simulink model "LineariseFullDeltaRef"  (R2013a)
settings: Solver=ode23tb  StartTime=0.0  StopTime=2  RelTol=1e-3
InitFcn:
  | SimParam.IC = SM2_InitCondConstrFnc(RawParam,IC);
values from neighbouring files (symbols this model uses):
  N = D(1)+(H4^2+H3^2)/H2^2-(E(1)*H4+F(1)*H3)/H2    [MGD.m]    (also in MGD2.m)
  RawParam = RobotParamGather(ParamLib)    [main_testIdentification3quad.m]    (also in DeltaModelMain_v2.m; main_TimeSimulation.m; MGI.m = y)
  s = -sign(imag(KGZ_fr_tmp))    [LinprogReguliOptimFunc_1.m]    (also in LinprogReguliOptimFunc_2.m; LinprogReguliOptimFunc_1 - Copie.m)
  X = varDefaultValue    [main_OptimModelParam1_subfunc1.m]    (also in main_OptimModelParam2_subfunc1.m; main_testIdentification3bis.m = [180e-6  370e-6         0.00182               0.95          ; main_testIdentification3tris.m = [180e-6 370e-6 0.00182 1 6.65e-3 0.0019 0.01 100  0.073  435; main_testIdentification3_ga_subfunc1.m)
  Y = fft(y(:,i),NFFT)/L    [fft_bis.m]    (also in MGI.m = -sin(phi(i))*x+cos(phi(i))*y)
  Z = z    [MGI.m]
undefined symbols (not defined in the file or in its folder): AxisID, kg, m, rad
libraries: sm_lib x29, SM2_ArmPartsLib x12, SM2_BallJointPartsLib x10, SM2_ForeArmPartsLib x6, nesl_utility x4, SM2_MotorPartsLib x3, SM2_FramePartsLib x1, SM2_ToolPartsLib x1

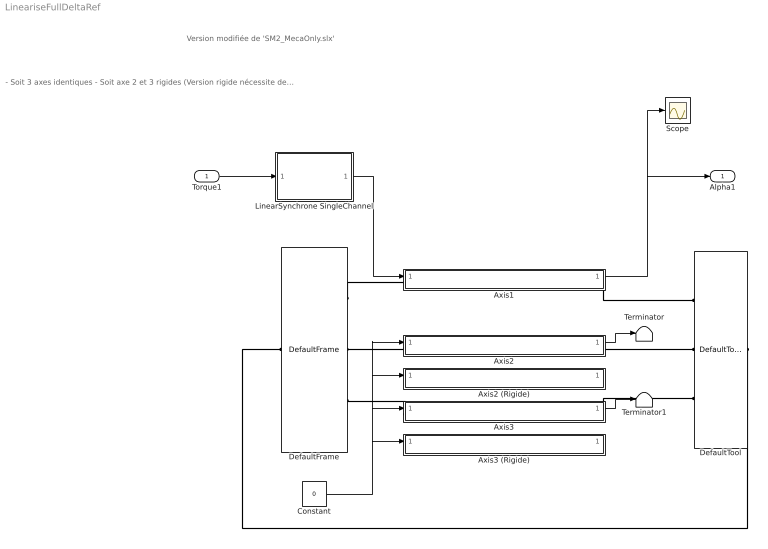
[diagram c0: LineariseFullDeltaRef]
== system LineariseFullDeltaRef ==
  note: - Soit 3 axes identiques - Soit axe 2 et 3 rigides (Version rigide nécessite des blocks non liés au libraries et des fonctions d'initialisaions indépendantes voir "local###_paramInitFnc()")
  note: Version modifiée de 'SM2_MecaOnly.slx'
  Torque1 : Inport
  Axis1 : Subsystem
  Axis2 : Subsystem
  Axis2 (Rigide) : Subsystem  Commented=on
  Axis3 : Subsystem
  Axis3 (Rigide) : Subsystem  Commented=on
  Constant : Constant  Value=0
  DefaultFrame : SM2_FramePartsLib/DefaultFrame
  DefaultTool : SM2_ToolPartsLib/DefaultTool
  LinearSynchrone SingleChannel : Subsystem  InitFcn=SimParam.Driver = driver_ParamInitFnc(RawParam,2);  VariantControl=driverVarLinearSynchrone
  Scope : Scope
  Terminator : Terminator
  Terminator1 : Terminator
  Alpha1 : Outport
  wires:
  Axis1/1(Alpha) -> Scope/1, Alpha1/1
  LinearSynchrone SingleChannel/1(Torque) -> Axis1/1(Torque)
  Torque1/1 -> LinearSynchrone SingleChannel/1(U)
  Axis3/1(Alpha) -> Terminator1/1
  Axis2/1(Alpha) -> Terminator/1
  Constant/1 -> Axis3 (Rigide)/1(Torque), Axis3/1(Torque), Axis2 (Rigide)/1(Torque), Axis2/1(Torque)
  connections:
  DefaultFrame/RConn1 -- Axis1/LConn1
  Axis1/RConn1 -- DefaultTool/RConn1
  DefaultTool/LConn1 -- DefaultFrame/LConn1
  Axis2/LConn1 -- DefaultFrame/RConn2
  Axis2/RConn1 -- DefaultTool/RConn2
  Axis3/LConn1 -- DefaultFrame/RConn3
  Axis3/RConn1 -- DefaultTool/RConn3

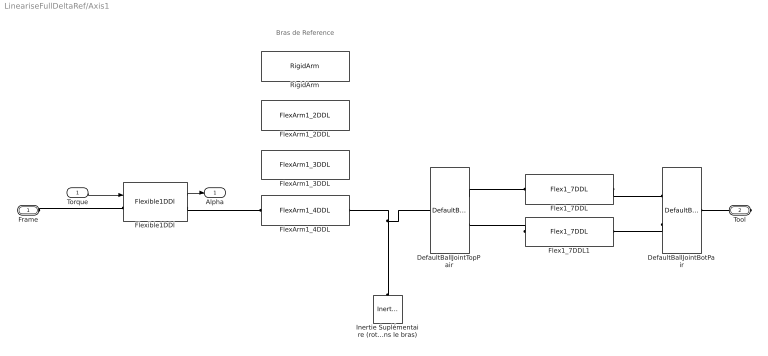
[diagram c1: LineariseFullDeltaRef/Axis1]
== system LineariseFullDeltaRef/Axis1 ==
  note: Bras de Reference
  Torque : Inport
  DefaultBallJointBotPair : SM2_BallJointPartsLib/DefaultBallJointBotPair
  DefaultBallJointTopPair : SM2_BallJointPartsLib/DefaultBallJointTopPair
  Flex1_7DDL : SM2_ForeArmPartsLib/Flex1_7DDL  VariantControl=foreArmVarFlex1_7ddl
  Flex1_7DDL1 : SM2_ForeArmPartsLib/Flex1_7DDL  VariantControl=foreArmVarFlex1_7ddl
  FlexArm1_2DDL : SM2_ArmPartsLib/FlexArm1_2DDL  Commented=on  VariantControl=armVarFlex1_2ddl
  FlexArm1_3DDL : SM2_ArmPartsLib/FlexArm1_3DDL  Commented=on  VariantControl=armVarFlex1_3ddl
  FlexArm1_4DDL : SM2_ArmPartsLib/FlexArm1_4DDL  VariantControl=armVarFlex1_4ddl
  Flexible1DDl : SM2_MotorPartsLib/Flexible1DDl  VariantControl=motorVarFlex1
  Inertie Suplémentaire (rotule déjà inclues dans le bras) : sm_lib/Body Elements/Inertia  InertiaType=Custom  Mass=SimParam.mend+1e-7  MassUnits=kg  CenterOfMass=[0 0 0]  CenterOfMassUnits=m  MomentsOfInertia=SimParam.Iend  MomentsOfInertiaUnits=kg*m^2  ProductsOfInertia=[0 0 0]  ProductsOfInertiaUnits=kg*m^2  BlockFunction=simmechanics.library.body_elements.inertia
  RigidArm : SM2_ArmPartsLib/RigidArm  Commented=on  VariantControl=armVarDefault
  Frame : PMIOPort  Port=1  Side=Left
  Tool : PMIOPort  Port=2  Side=Right
  Alpha : Outport
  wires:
  Torque/1 -> Flexible1DDl/1
  Flexible1DDl/1 -> Alpha/1
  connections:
  Frame/RConn1 -- Flexible1DDl/LConn1
  Flexible1DDl/RConn1 -- FlexArm1_4DDL/LConn1
  Inertie Suplémentaire (rotule déjà inclues dans le bras)/RConn1 -- FlexArm1_4DDL/RConn1 -- DefaultBallJointTopPair/RConn1
  Flex1_7DDL1/LConn1 -- DefaultBallJointTopPair/LConn2
  DefaultBallJointTopPair/LConn1 -- Flex1_7DDL/LConn1
  Flex1_7DDL/RConn1 -- DefaultBallJointBotPair/LConn1
  DefaultBallJointBotPair/LConn2 -- Flex1_7DDL1/RConn1
  Tool/RConn1 -- DefaultBallJointBotPair/RConn1

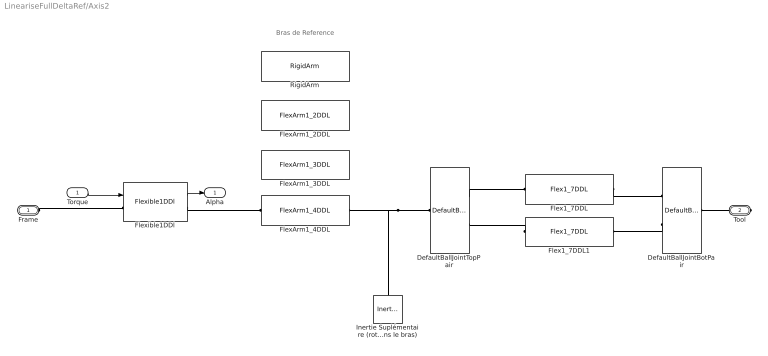
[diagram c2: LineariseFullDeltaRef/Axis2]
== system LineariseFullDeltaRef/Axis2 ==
  note: Bras de Reference
  Torque : Inport
  DefaultBallJointBotPair : SM2_BallJointPartsLib/DefaultBallJointBotPair
  DefaultBallJointTopPair : SM2_BallJointPartsLib/DefaultBallJointTopPair
  Flex1_7DDL : SM2_ForeArmPartsLib/Flex1_7DDL  VariantControl=foreArmVarFlex1_7ddl
  Flex1_7DDL1 : SM2_ForeArmPartsLib/Flex1_7DDL  VariantControl=foreArmVarFlex1_7ddl
  FlexArm1_2DDL : SM2_ArmPartsLib/FlexArm1_2DDL  Commented=on  VariantControl=armVarFlex1_2ddl
  FlexArm1_3DDL : SM2_ArmPartsLib/FlexArm1_3DDL  Commented=on  VariantControl=armVarFlex1_3ddl
  FlexArm1_4DDL : SM2_ArmPartsLib/FlexArm1_4DDL  VariantControl=armVarFlex1_4ddl
  Flexible1DDl : SM2_MotorPartsLib/Flexible1DDl  VariantControl=motorVarFlex1
  Inertie Suplémentaire (rotule déjà inclues dans le bras) : sm_lib/Body Elements/Inertia  InertiaType=Custom  Mass=SimParam.mend+1e-7  MassUnits=kg  CenterOfMass=[0 0 0]  CenterOfMassUnits=m  MomentsOfInertia=SimParam.Iend  MomentsOfInertiaUnits=kg*m^2  ProductsOfInertia=[0 0 0]  ProductsOfInertiaUnits=kg*m^2  BlockFunction=simmechanics.library.body_elements.inertia
  RigidArm : SM2_ArmPartsLib/RigidArm  Commented=on  VariantControl=armVarDefault
  Frame : PMIOPort  Port=1  Side=Left
  Tool : PMIOPort  Port=2  Side=Right
  Alpha : Outport
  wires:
  Torque/1 -> Flexible1DDl/1
  Flexible1DDl/1 -> Alpha/1
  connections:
  Frame/RConn1 -- Flexible1DDl/LConn1
  Flexible1DDl/RConn1 -- FlexArm1_4DDL/LConn1
  DefaultBallJointTopPair/RConn1 -- Inertie Suplémentaire (rotule déjà inclues dans le bras)/RConn1 -- FlexArm1_4DDL/RConn1
  Flex1_7DDL1/LConn1 -- DefaultBallJointTopPair/LConn2
  DefaultBallJointTopPair/LConn1 -- Flex1_7DDL/LConn1
  Flex1_7DDL/RConn1 -- DefaultBallJointBotPair/LConn1
  DefaultBallJointBotPair/LConn2 -- Flex1_7DDL1/RConn1
  Tool/RConn1 -- DefaultBallJointBotPair/RConn1

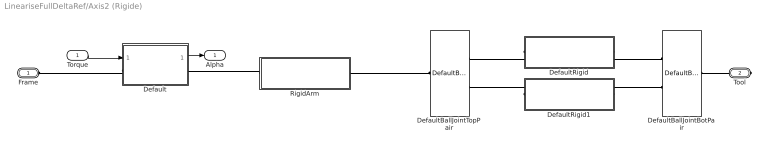
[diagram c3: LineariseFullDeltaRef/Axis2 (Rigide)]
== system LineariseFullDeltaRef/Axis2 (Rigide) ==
  Torque : Inport
  Default : Subsystem  InitFcn=SimParam.Motor2=localRigidMotor_paramInitFnc(RawParam,IC);  VariantControl=motorVarDefault
  DefaultBallJointBotPair : SM2_BallJointPartsLib/DefaultBallJointBotPair
  DefaultBallJointTopPair : SM2_BallJointPartsLib/DefaultBallJointTopPair
  DefaultRigid : Subsystem  InitFcn=SimParam.ForeArm2 = localRigidForeArm_paramInitFnc(RawParam,0);  VariantControl=foreArmVarDefault
  DefaultRigid1 : Subsystem  InitFcn=SimParam.ForeArm2 = localRigidForeArm_paramInitFnc(RawParam,0);  VariantControl=foreArmVarDefault
  RigidArm : Subsystem  InitFcn=SimParam.Arm2=localRigidArm_paramInitFnc(RawParam,0);  VariantControl=armVarDefault
  Frame : PMIOPort  Port=1  Side=Left
  Tool : PMIOPort  Port=2  Side=Right
  Alpha : Outport
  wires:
  Torque/1 -> Default/1(Torque)
  Default/1(Alpha) -> Alpha/1
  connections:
  Default/LConn1 -- Frame/RConn1
  RigidArm/LConn1 -- Default/RConn1
  RigidArm/RConn1 -- DefaultBallJointTopPair/RConn1
  DefaultRigid1/LConn1 -- DefaultBallJointTopPair/LConn2
  DefaultRigid/LConn1 -- DefaultBallJointTopPair/LConn1
  DefaultRigid/RConn1 -- DefaultBallJointBotPair/LConn1
  DefaultRigid1/RConn1 -- DefaultBallJointBotPair/LConn2
  Tool/RConn1 -- DefaultBallJointBotPair/RConn1

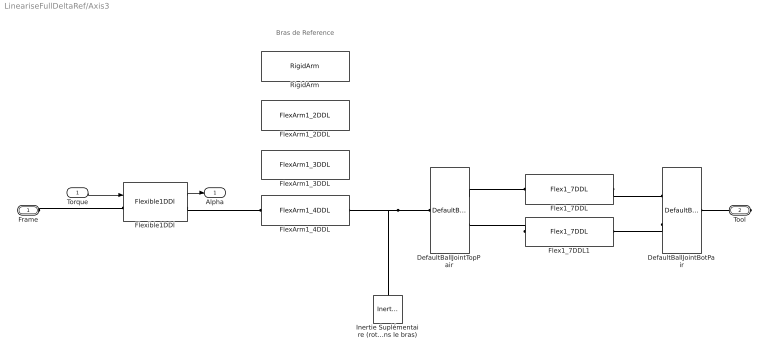
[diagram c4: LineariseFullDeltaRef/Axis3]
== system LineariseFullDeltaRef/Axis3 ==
  note: Bras de Reference
  Torque : Inport
  DefaultBallJointBotPair : SM2_BallJointPartsLib/DefaultBallJointBotPair
  DefaultBallJointTopPair : SM2_BallJointPartsLib/DefaultBallJointTopPair
  Flex1_7DDL : SM2_ForeArmPartsLib/Flex1_7DDL  VariantControl=foreArmVarFlex1_7ddl
  Flex1_7DDL1 : SM2_ForeArmPartsLib/Flex1_7DDL  VariantControl=foreArmVarFlex1_7ddl
  FlexArm1_2DDL : SM2_ArmPartsLib/FlexArm1_2DDL  Commented=on  VariantControl=armVarFlex1_2ddl
  FlexArm1_3DDL : SM2_ArmPartsLib/FlexArm1_3DDL  Commented=on  VariantControl=armVarFlex1_3ddl
  FlexArm1_4DDL : SM2_ArmPartsLib/FlexArm1_4DDL  VariantControl=armVarFlex1_4ddl
  Flexible1DDl : SM2_MotorPartsLib/Flexible1DDl  VariantControl=motorVarFlex1
  Inertie Suplémentaire (rotule déjà inclues dans le bras) : sm_lib/Body Elements/Inertia  InertiaType=Custom  Mass=SimParam.mend+1e-7  MassUnits=kg  CenterOfMass=[0 0 0]  CenterOfMassUnits=m  MomentsOfInertia=SimParam.Iend  MomentsOfInertiaUnits=kg*m^2  ProductsOfInertia=[0 0 0]  ProductsOfInertiaUnits=kg*m^2  BlockFunction=simmechanics.library.body_elements.inertia
  RigidArm : SM2_ArmPartsLib/RigidArm  Commented=on  VariantControl=armVarDefault
  Frame : PMIOPort  Port=1  Side=Left
  Tool : PMIOPort  Port=2  Side=Right
  Alpha : Outport
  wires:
  Torque/1 -> Flexible1DDl/1
  Flexible1DDl/1 -> Alpha/1
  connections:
  Frame/RConn1 -- Flexible1DDl/LConn1
  Flexible1DDl/RConn1 -- FlexArm1_4DDL/LConn1
  DefaultBallJointTopPair/RConn1 -- Inertie Suplémentaire (rotule déjà inclues dans le bras)/RConn1 -- FlexArm1_4DDL/RConn1
  Flex1_7DDL1/LConn1 -- DefaultBallJointTopPair/LConn2
  DefaultBallJointTopPair/LConn1 -- Flex1_7DDL/LConn1
  Flex1_7DDL/RConn1 -- DefaultBallJointBotPair/LConn1
  DefaultBallJointBotPair/LConn2 -- Flex1_7DDL1/RConn1
  Tool/RConn1 -- DefaultBallJointBotPair/RConn1

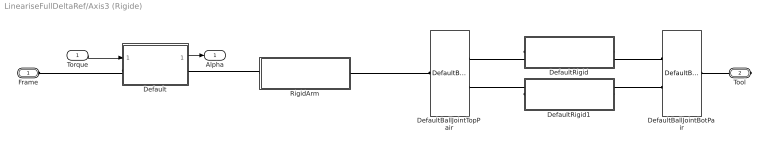
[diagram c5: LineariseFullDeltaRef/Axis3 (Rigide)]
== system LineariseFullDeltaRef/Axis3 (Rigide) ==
  Torque : Inport
  Default : Subsystem  InitFcn=SimParam.Motor2=localRigidMotor_paramInitFnc(RawParam,IC);  VariantControl=motorVarDefault
  DefaultBallJointBotPair : SM2_BallJointPartsLib/DefaultBallJointBotPair
  DefaultBallJointTopPair : SM2_BallJointPartsLib/DefaultBallJointTopPair
  DefaultRigid : Subsystem  InitFcn=SimParam.ForeArm2 = localRigidForeArm_paramInitFnc(RawParam,0);  VariantControl=foreArmVarDefault
  DefaultRigid1 : Subsystem  InitFcn=SimParam.ForeArm2 = localRigidForeArm_paramInitFnc(RawParam,0);  VariantControl=foreArmVarDefault
  RigidArm : Subsystem  InitFcn=SimParam.Arm2=localRigidArm_paramInitFnc(RawParam,0);  VariantControl=armVarDefault
  Frame : PMIOPort  Port=1  Side=Left
  Tool : PMIOPort  Port=2  Side=Right
  Alpha : Outport
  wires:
  Torque/1 -> Default/1(Torque)
  Default/1(Alpha) -> Alpha/1
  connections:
  Default/LConn1 -- Frame/RConn1
  RigidArm/LConn1 -- Default/RConn1
  RigidArm/RConn1 -- DefaultBallJointTopPair/RConn1
  DefaultRigid1/LConn1 -- DefaultBallJointTopPair/LConn2
  DefaultRigid/LConn1 -- DefaultBallJointTopPair/LConn1
  DefaultRigid/RConn1 -- DefaultBallJointBotPair/LConn1
  DefaultRigid1/RConn1 -- DefaultBallJointBotPair/LConn2
  Tool/RConn1 -- DefaultBallJointBotPair/RConn1

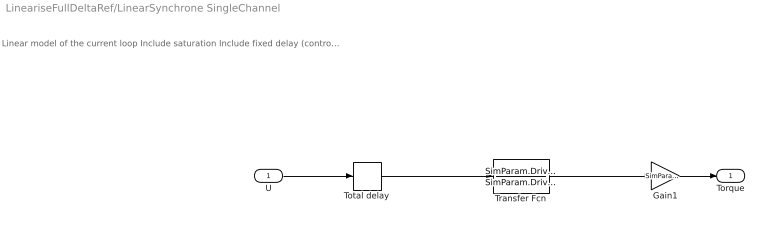
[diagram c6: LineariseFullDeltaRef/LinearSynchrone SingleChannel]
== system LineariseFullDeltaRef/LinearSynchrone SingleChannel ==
  note: Linear model of the current loop Include saturation Include fixed delay (control delay + driver delay + 0.5*driver sample periode if assynchonous)
  U : Inport
  Gain1 : Gain  Gain=SimParam.Driver.GRelScale
  Total delay : TransportDelay  DelayTime=SimParam.Driver.tau  BufferSize=10000
  Transfer Fcn : TransferFcn  Numerator=SimParam.Driver.TfNum  Denominator=SimParam.Driver.TfDen
  Torque : Outport
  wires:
  Total delay/1 -> Transfer Fcn/1
  Gain1/1 -> Torque/1
  U/1 -> Total delay/1
  Transfer Fcn/1 -> Gain1/1

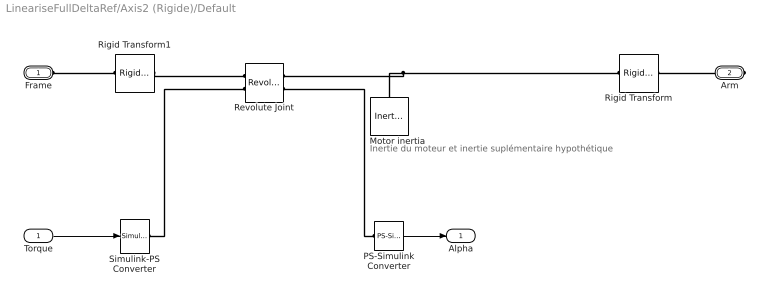
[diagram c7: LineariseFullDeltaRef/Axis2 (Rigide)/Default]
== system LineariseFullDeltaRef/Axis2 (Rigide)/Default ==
  note: Inertie du moteur et inertie suplémentaire hypothétique
  Torque : Inport
  Motor inertia : sm_lib/Body Elements/Inertia  InertiaType=Custom  Mass=1  MassUnits=kg  CenterOfMass=[0 0 0]  CenterOfMassUnits=m  MomentsOfInertia=(SimParam.Motor2.I+SimParam.Motor2.ISup).*[1 1 1]  MomentsOfInertiaUnits=kg*m^2  ProductsOfInertia=[0 0 0]  ProductsOfInertiaUnits=kg*m^2  BlockFunction=simmechanics.library.body_elements.inertia
  PS-Simulink Converter : nesl_utility/PS-Simulink Converter  PhysicalDomain=network_engine_domain  SubClassName=ps_output  LeftPortType=input  RightPortType=output  PseudoPeriodic=off  Frequencies=[]  Unit=1  AffineConversion=off
  Revolute Joint : sm_lib/Joints/Revolute Joint  SenseConstraintForceX=off  SenseConstraintForceY=off  SenseConstraintForceZ=off  SenseConstraintTorqueX=off  SenseConstraintTorqueY=off  SenseConstraintTorqueZ=off  ConstraintWrenchDir=FollowerOnBase  ConstraintWrenchFrame=BaseFrame  EquilibriumPosition=SimParam.Motor2.Alpha(AxisID)  EquilibriumPositionUnits=rad  SpringStiffness=SimParam.Motor2.kSup  SpringStiffnessUnits=N*m/rad  DampingCoefficient=SimParam.Motor2.c  DampingCoefficientUnits=N*m/(rad/s)  ActuationMode=TorqueForceActuation  SensePosition=on  SenseVelocity=off  SenseAcceleration=off  SenseTorqueForce=off  PositionTargetValue=SimParam.Motor2.Alpha(AxisID)  PositionTargetValueUnits=rad  PositionTargetSpecify=on  PositionTargetPriority=High  VelocityTargetValue=0  VelocityTargetValueUnits=rad/s  VelocityTargetSpecify=on  VelocityTargetPriority=High  BlockFunction=simmechanics.library.joints.revolute_joint
  Rigid Transform : sm_lib/Frames and  Transforms/Rigid  Transform  TranslationMethod=None  TranslationLengthUnit=m  TranslationStandardAxis=+Z  TranslationStandardOffset=0  TranslationCartesianOffset=[0 0 0]  TranslationROffset=0.2  TranslationROffsetUnits=m  TranslationZOffset=0  TranslationZOffsetUnits=m  TranslationThetaOffset=0  TranslationThetaOffsetUnits=deg  RotationMethod=AlignedAxes  RotationAngleUnits=rad  RotationStandardAxis=+Y  RotationAngle=0.2  RotationArbitraryAxis=[0 0 1]  FollAlignAxisA=+Y  BaseAlignAxisA=+Z  FollAlignAxisB=+X  BaseAlignAxisB=+X  BlockFunction=simmechanics.library.frames_transforms.rigid_transform
  Rigid Transform1 : sm_lib/Frames and  Transforms/Rigid  Transform  TranslationMethod=None  TranslationLengthUnit=m  TranslationStandardAxis=+Z  TranslationStandardOffset=0  TranslationCartesianOffset=[0 0 0]  TranslationROffset=0.2  TranslationROffsetUnits=m  TranslationZOffset=0  TranslationZOffsetUnits=m  TranslationThetaOffset=0  TranslationThetaOffsetUnits=deg  RotationMethod=AlignedAxes  RotationAngleUnits=rad  RotationStandardAxis=+Y  RotationAngle=0.2  RotationArbitraryAxis=[0 0 1]  FollAlignAxisA=+Z  BaseAlignAxisA=+Y  FollAlignAxisB=+X  BaseAlignAxisB=+X  BlockFunction=simmechanics.library.frames_transforms.rigid_transform
  Simulink-PS Converter : nesl_utility/Simulink-PS Converter  PhysicalDomain=network_engine_domain  SubClassName=ps_input  LeftPortType=input  RightPortType=output  PseudoPeriodic=off  Frequencies=[]  NoiseDistribution=none  NoiseParameters=[]  Unit=1  AffineConversion=off  InputFiltering=off  SimscapeFilterOrder=1  InputFilterTimeConstant=0.001  UdotUserProvided=1
  Frame : PMIOPort  Port=1  Side=Left
  Arm : PMIOPort  Port=2  Side=Right
  Alpha : Outport
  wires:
  Torque/1 -> Simulink-PS Converter/1
  PS-Simulink Converter/1 -> Alpha/1
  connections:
  Arm/RConn1 -- Rigid Transform/RConn1
  Rigid Transform1/LConn1 -- Frame/RConn1
  PS-Simulink Converter/LConn1 -- Revolute Joint/RConn2
  Rigid Transform/LConn1 -- Revolute Joint/RConn1 -- Motor inertia/RConn1
  Rigid Transform1/RConn1 -- Revolute Joint/LConn1
  Simulink-PS Converter/RConn1 -- Revolute Joint/LConn2

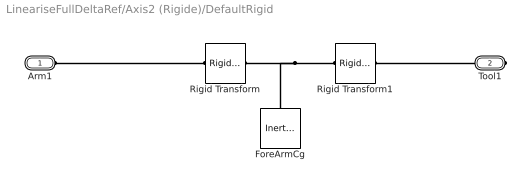
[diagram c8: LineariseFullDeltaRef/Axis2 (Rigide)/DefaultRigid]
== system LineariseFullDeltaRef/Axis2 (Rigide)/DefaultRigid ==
  ForeArmCg : sm_lib/Body Elements/Inertia  InertiaType=Custom  Mass=SimParam.ForeArm2.m  MassUnits=kg  CenterOfMass=[0 0 0]  CenterOfMassUnits=m  MomentsOfInertia=SimParam.ForeArm2.I  MomentsOfInertiaUnits=kg*m^2  ProductsOfInertia=[0 0 0]  ProductsOfInertiaUnits=kg*m^2  BlockFunction=simmechanics.library.body_elements.inertia
  Rigid Transform : sm_lib/Frames and  Transforms/Rigid  Transform  TranslationMethod=Cartesian  TranslationLengthUnit=m  TranslationStandardAxis=+Z  TranslationStandardOffset=0  TranslationCartesianOffset=[SimParam.ForeArm2.lcg 0 0]  TranslationROffset=0  TranslationROffsetUnits=m  TranslationZOffset=0  TranslationZOffsetUnits=m  TranslationThetaOffset=0  TranslationThetaOffsetUnits=deg  RotationMethod=None  RotationAngleUnits=deg  RotationStandardAxis=+Z  RotationAngle=0  RotationArbitraryAxis=[0 0 1]  FollAlignAxisA=+X  BaseAlignAxisA=+Y  FollAlignAxisB=+Y  BaseAlignAxisB=+Z  BlockFunction=simmechanics.library.frames_transforms.rigid_transform
  Rigid Transform1 : sm_lib/Frames and  Transforms/Rigid  Transform  TranslationMethod=Cartesian  TranslationLengthUnit=m  TranslationStandardAxis=+Z  TranslationStandardOffset=0  TranslationCartesianOffset=[SimParam.ForeArm2.l-SimParam.ForeArm2.lcg 0 0]  TranslationROffset=0  TranslationROffsetUnits=m  TranslationZOffset=0  TranslationZOffsetUnits=m  TranslationThetaOffset=0  TranslationThetaOffsetUnits=deg  RotationMethod=AlignedAxes  RotationAngleUnits=deg  RotationStandardAxis=+Z  RotationAngle=0  RotationArbitraryAxis=[0 0 1]  FollAlignAxisA=-Z  BaseAlignAxisA=+X  FollAlignAxisB=+Y  BaseAlignAxisB=+Y  BlockFunction=simmechanics.library.frames_transforms.rigid_transform
  Arm1 : PMIOPort  Port=1  Side=Left
  Tool1 : PMIOPort  Port=2  Side=Right
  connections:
  Tool1/RConn1 -- Rigid Transform1/RConn1
  Arm1/RConn1 -- Rigid Transform/LConn1
  Rigid Transform1/LConn1 -- Rigid Transform/RConn1 -- ForeArmCg/RConn1

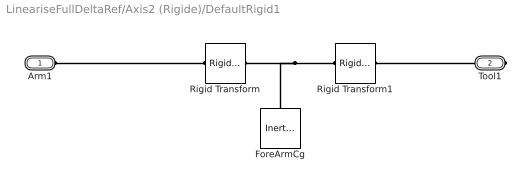
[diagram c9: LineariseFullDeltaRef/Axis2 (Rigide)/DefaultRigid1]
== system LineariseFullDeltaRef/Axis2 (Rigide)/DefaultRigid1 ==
  ForeArmCg : sm_lib/Body Elements/Inertia  InertiaType=Custom  Mass=SimParam.ForeArm2.m  MassUnits=kg  CenterOfMass=[0 0 0]  CenterOfMassUnits=m  MomentsOfInertia=SimParam.ForeArm2.I  MomentsOfInertiaUnits=kg*m^2  ProductsOfInertia=[0 0 0]  ProductsOfInertiaUnits=kg*m^2  BlockFunction=simmechanics.library.body_elements.inertia
  Rigid Transform : sm_lib/Frames and  Transforms/Rigid  Transform  TranslationMethod=Cartesian  TranslationLengthUnit=m  TranslationStandardAxis=+Z  TranslationStandardOffset=0  TranslationCartesianOffset=[SimParam.ForeArm2.lcg 0 0]  TranslationROffset=0  TranslationROffsetUnits=m  TranslationZOffset=0  TranslationZOffsetUnits=m  TranslationThetaOffset=0  TranslationThetaOffsetUnits=deg  RotationMethod=None  RotationAngleUnits=deg  RotationStandardAxis=+Z  RotationAngle=0  RotationArbitraryAxis=[0 0 1]  FollAlignAxisA=+X  BaseAlignAxisA=+Y  FollAlignAxisB=+Y  BaseAlignAxisB=+Z  BlockFunction=simmechanics.library.frames_transforms.rigid_transform
  Rigid Transform1 : sm_lib/Frames and  Transforms/Rigid  Transform  TranslationMethod=Cartesian  TranslationLengthUnit=m  TranslationStandardAxis=+Z  TranslationStandardOffset=0  TranslationCartesianOffset=[SimParam.ForeArm2.l-SimParam.ForeArm2.lcg 0 0]  TranslationROffset=0  TranslationROffsetUnits=m  TranslationZOffset=0  TranslationZOffsetUnits=m  TranslationThetaOffset=0  TranslationThetaOffsetUnits=deg  RotationMethod=AlignedAxes  RotationAngleUnits=deg  RotationStandardAxis=+Z  RotationAngle=0  RotationArbitraryAxis=[0 0 1]  FollAlignAxisA=-Z  BaseAlignAxisA=+X  FollAlignAxisB=+Y  BaseAlignAxisB=+Y  BlockFunction=simmechanics.library.frames_transforms.rigid_transform
  Arm1 : PMIOPort  Port=1  Side=Left
  Tool1 : PMIOPort  Port=2  Side=Right
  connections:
  Tool1/RConn1 -- Rigid Transform1/RConn1
  Arm1/RConn1 -- Rigid Transform/LConn1
  Rigid Transform1/LConn1 -- Rigid Transform/RConn1 -- ForeArmCg/RConn1

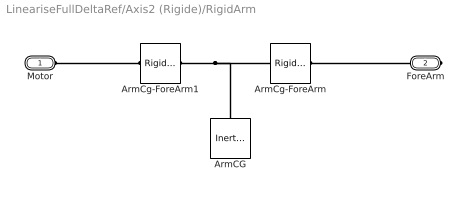
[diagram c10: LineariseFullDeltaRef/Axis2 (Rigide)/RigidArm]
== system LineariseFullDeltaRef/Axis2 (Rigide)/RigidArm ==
  ArmCG : sm_lib/Body Elements/Inertia  InertiaType=Custom  Mass=SimParam.Arm2.m  MassUnits=kg  CenterOfMass=[0 0 0]  CenterOfMassUnits=m  MomentsOfInertia=SimParam.Arm2.I'  MomentsOfInertiaUnits=kg*m^2  ProductsOfInertia=[0 0 0]  ProductsOfInertiaUnits=kg*m^2  BlockFunction=simmechanics.library.body_elements.inertia
  ArmCg-ForeArm : sm_lib/Frames and  Transforms/Rigid  Transform  TranslationMethod=Cartesian  TranslationLengthUnit=m  TranslationStandardAxis=+Z  TranslationStandardOffset=0  TranslationCartesianOffset=[SimParam.Arm2.l-SimParam.Arm2.lcg 0 0]  TranslationROffset=0  TranslationROffsetUnits=m  TranslationZOffset=0  TranslationZOffsetUnits=m  TranslationThetaOffset=0  TranslationThetaOffsetUnits=deg  RotationMethod=None  RotationAngleUnits=deg  RotationStandardAxis=+Z  RotationAngle=0  RotationArbitraryAxis=[0 0 1]  FollAlignAxisA=+X  BaseAlignAxisA=+Y  FollAlignAxisB=+Y  BaseAlignAxisB=+Z  BlockFunction=simmechanics.library.frames_transforms.rigid_transform
  ArmCg-ForeArm1 : sm_lib/Frames and  Transforms/Rigid  Transform  TranslationMethod=Cartesian  TranslationLengthUnit=m  TranslationStandardAxis=+Z  TranslationStandardOffset=0  TranslationCartesianOffset=[SimParam.Arm2.lcg 0 0]  TranslationROffset=0  TranslationROffsetUnits=m  TranslationZOffset=0  TranslationZOffsetUnits=m  TranslationThetaOffset=0  TranslationThetaOffsetUnits=deg  RotationMethod=None  RotationAngleUnits=deg  RotationStandardAxis=+Z  RotationAngle=0  RotationArbitraryAxis=[0 0 1]  FollAlignAxisA=+X  BaseAlignAxisA=+Y  FollAlignAxisB=+Y  BaseAlignAxisB=+Z  BlockFunction=simmechanics.library.frames_transforms.rigid_transform
  Motor : PMIOPort  Port=1  Side=Left
  ForeArm : PMIOPort  Port=2  Side=Right
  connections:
  ArmCg-ForeArm1/LConn1 -- Motor/RConn1
  ForeArm/RConn1 -- ArmCg-ForeArm/RConn1
  ArmCg-ForeArm1/RConn1 -- ArmCG/RConn1 -- ArmCg-ForeArm/LConn1

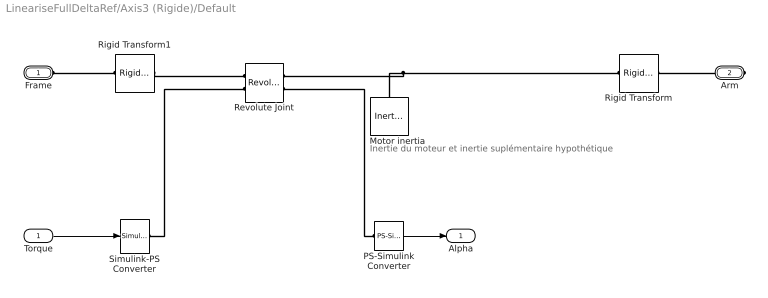
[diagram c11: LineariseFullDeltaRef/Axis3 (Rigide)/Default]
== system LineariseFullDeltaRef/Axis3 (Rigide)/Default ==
  note: Inertie du moteur et inertie suplémentaire hypothétique
  Torque : Inport
  Motor inertia : sm_lib/Body Elements/Inertia  InertiaType=Custom  Mass=1  MassUnits=kg  CenterOfMass=[0 0 0]  CenterOfMassUnits=m  MomentsOfInertia=(SimParam.Motor2.I+SimParam.Motor2.ISup).*[1 1 1]  MomentsOfInertiaUnits=kg*m^2  ProductsOfInertia=[0 0 0]  ProductsOfInertiaUnits=kg*m^2  BlockFunction=simmechanics.library.body_elements.inertia
  PS-Simulink Converter : nesl_utility/PS-Simulink Converter  PhysicalDomain=network_engine_domain  SubClassName=ps_output  LeftPortType=input  RightPortType=output  PseudoPeriodic=off  Frequencies=[]  Unit=1  AffineConversion=off
  Revolute Joint : sm_lib/Joints/Revolute Joint  SenseConstraintForceX=off  SenseConstraintForceY=off  SenseConstraintForceZ=off  SenseConstraintTorqueX=off  SenseConstraintTorqueY=off  SenseConstraintTorqueZ=off  ConstraintWrenchDir=FollowerOnBase  ConstraintWrenchFrame=BaseFrame  EquilibriumPosition=SimParam.Motor2.Alpha(AxisID)  EquilibriumPositionUnits=rad  SpringStiffness=SimParam.Motor2.kSup  SpringStiffnessUnits=N*m/rad  DampingCoefficient=SimParam.Motor2.c  DampingCoefficientUnits=N*m/(rad/s)  ActuationMode=TorqueForceActuation  SensePosition=on  SenseVelocity=off  SenseAcceleration=off  SenseTorqueForce=off  PositionTargetValue=SimParam.Motor2.Alpha(AxisID)  PositionTargetValueUnits=rad  PositionTargetSpecify=on  PositionTargetPriority=High  VelocityTargetValue=0  VelocityTargetValueUnits=rad/s  VelocityTargetSpecify=on  VelocityTargetPriority=High  BlockFunction=simmechanics.library.joints.revolute_joint
  Rigid Transform : sm_lib/Frames and  Transforms/Rigid  Transform  TranslationMethod=None  TranslationLengthUnit=m  TranslationStandardAxis=+Z  TranslationStandardOffset=0  TranslationCartesianOffset=[0 0 0]  TranslationROffset=0.2  TranslationROffsetUnits=m  TranslationZOffset=0  TranslationZOffsetUnits=m  TranslationThetaOffset=0  TranslationThetaOffsetUnits=deg  RotationMethod=AlignedAxes  RotationAngleUnits=rad  RotationStandardAxis=+Y  RotationAngle=0.2  RotationArbitraryAxis=[0 0 1]  FollAlignAxisA=+Y  BaseAlignAxisA=+Z  FollAlignAxisB=+X  BaseAlignAxisB=+X  BlockFunction=simmechanics.library.frames_transforms.rigid_transform
  Rigid Transform1 : sm_lib/Frames and  Transforms/Rigid  Transform  TranslationMethod=None  TranslationLengthUnit=m  TranslationStandardAxis=+Z  TranslationStandardOffset=0  TranslationCartesianOffset=[0 0 0]  TranslationROffset=0.2  TranslationROffsetUnits=m  TranslationZOffset=0  TranslationZOffsetUnits=m  TranslationThetaOffset=0  TranslationThetaOffsetUnits=deg  RotationMethod=AlignedAxes  RotationAngleUnits=rad  RotationStandardAxis=+Y  RotationAngle=0.2  RotationArbitraryAxis=[0 0 1]  FollAlignAxisA=+Z  BaseAlignAxisA=+Y  FollAlignAxisB=+X  BaseAlignAxisB=+X  BlockFunction=simmechanics.library.frames_transforms.rigid_transform
  Simulink-PS Converter : nesl_utility/Simulink-PS Converter  PhysicalDomain=network_engine_domain  SubClassName=ps_input  LeftPortType=input  RightPortType=output  PseudoPeriodic=off  Frequencies=[]  NoiseDistribution=none  NoiseParameters=[]  Unit=1  AffineConversion=off  InputFiltering=off  SimscapeFilterOrder=1  InputFilterTimeConstant=0.001  UdotUserProvided=1
  Frame : PMIOPort  Port=1  Side=Left
  Arm : PMIOPort  Port=2  Side=Right
  Alpha : Outport
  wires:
  Torque/1 -> Simulink-PS Converter/1
  PS-Simulink Converter/1 -> Alpha/1
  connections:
  Arm/RConn1 -- Rigid Transform/RConn1
  Rigid Transform1/LConn1 -- Frame/RConn1
  PS-Simulink Converter/LConn1 -- Revolute Joint/RConn2
  Rigid Transform/LConn1 -- Revolute Joint/RConn1 -- Motor inertia/RConn1
  Rigid Transform1/RConn1 -- Revolute Joint/LConn1
  Simulink-PS Converter/RConn1 -- Revolute Joint/LConn2

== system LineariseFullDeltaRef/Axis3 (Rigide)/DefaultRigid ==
  ForeArmCg : sm_lib/Body Elements/Inertia  InertiaType=Custom  Mass=SimParam.ForeArm2.m  MassUnits=kg  CenterOfMass=[0 0 0]  CenterOfMassUnits=m  MomentsOfInertia=SimParam.ForeArm2.I  MomentsOfInertiaUnits=kg*m^2  ProductsOfInertia=[0 0 0]  ProductsOfInertiaUnits=kg*m^2  BlockFunction=simmechanics.library.body_elements.inertia
  Rigid Transform : sm_lib/Frames and  Transforms/Rigid  Transform  TranslationMethod=Cartesian  TranslationLengthUnit=m  TranslationStandardAxis=+Z  TranslationStandardOffset=0  TranslationCartesianOffset=[SimParam.ForeArm2.lcg 0 0]  TranslationROffset=0  TranslationROffsetUnits=m  TranslationZOffset=0  TranslationZOffsetUnits=m  TranslationThetaOffset=0  TranslationThetaOffsetUnits=deg  RotationMethod=None  RotationAngleUnits=deg  RotationStandardAxis=+Z  RotationAngle=0  RotationArbitraryAxis=[0 0 1]  FollAlignAxisA=+X  BaseAlignAxisA=+Y  FollAlignAxisB=+Y  BaseAlignAxisB=+Z  BlockFunction=simmechanics.library.frames_transforms.rigid_transform
  Rigid Transform1 : sm_lib/Frames and  Transforms/Rigid  Transform  TranslationMethod=Cartesian  TranslationLengthUnit=m  TranslationStandardAxis=+Z  TranslationStandardOffset=0  TranslationCartesianOffset=[SimParam.ForeArm2.l-SimParam.ForeArm2.lcg 0 0]  TranslationROffset=0  TranslationROffsetUnits=m  TranslationZOffset=0  TranslationZOffsetUnits=m  TranslationThetaOffset=0  TranslationThetaOffsetUnits=deg  RotationMethod=AlignedAxes  RotationAngleUnits=deg  RotationStandardAxis=+Z  RotationAngle=0  RotationArbitraryAxis=[0 0 1]  FollAlignAxisA=-Z  BaseAlignAxisA=+X  FollAlignAxisB=+Y  BaseAlignAxisB=+Y  BlockFunction=simmechanics.library.frames_transforms.rigid_transform
  Arm1 : PMIOPort  Port=1  Side=Left
  Tool1 : PMIOPort  Port=2  Side=Right
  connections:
  Tool1/RConn1 -- Rigid Transform1/RConn1
  Arm1/RConn1 -- Rigid Transform/LConn1
  Rigid Transform1/LConn1 -- Rigid Transform/RConn1 -- ForeArmCg/RConn1

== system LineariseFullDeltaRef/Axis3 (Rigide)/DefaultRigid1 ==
  ForeArmCg : sm_lib/Body Elements/Inertia  InertiaType=Custom  Mass=SimParam.ForeArm2.m  MassUnits=kg  CenterOfMass=[0 0 0]  CenterOfMassUnits=m  MomentsOfInertia=SimParam.ForeArm2.I  MomentsOfInertiaUnits=kg*m^2  ProductsOfInertia=[0 0 0]  ProductsOfInertiaUnits=kg*m^2  BlockFunction=simmechanics.library.body_elements.inertia
  Rigid Transform : sm_lib/Frames and  Transforms/Rigid  Transform  TranslationMethod=Cartesian  TranslationLengthUnit=m  TranslationStandardAxis=+Z  TranslationStandardOffset=0  TranslationCartesianOffset=[SimParam.ForeArm2.lcg 0 0]  TranslationROffset=0  TranslationROffsetUnits=m  TranslationZOffset=0  TranslationZOffsetUnits=m  TranslationThetaOffset=0  TranslationThetaOffsetUnits=deg  RotationMethod=None  RotationAngleUnits=deg  RotationStandardAxis=+Z  RotationAngle=0  RotationArbitraryAxis=[0 0 1]  FollAlignAxisA=+X  BaseAlignAxisA=+Y  FollAlignAxisB=+Y  BaseAlignAxisB=+Z  BlockFunction=simmechanics.library.frames_transforms.rigid_transform
  Rigid Transform1 : sm_lib/Frames and  Transforms/Rigid  Transform  TranslationMethod=Cartesian  TranslationLengthUnit=m  TranslationStandardAxis=+Z  TranslationStandardOffset=0  TranslationCartesianOffset=[SimParam.ForeArm2.l-SimParam.ForeArm2.lcg 0 0]  TranslationROffset=0  TranslationROffsetUnits=m  TranslationZOffset=0  TranslationZOffsetUnits=m  TranslationThetaOffset=0  TranslationThetaOffsetUnits=deg  RotationMethod=AlignedAxes  RotationAngleUnits=deg  RotationStandardAxis=+Z  RotationAngle=0  RotationArbitraryAxis=[0 0 1]  FollAlignAxisA=-Z  BaseAlignAxisA=+X  FollAlignAxisB=+Y  BaseAlignAxisB=+Y  BlockFunction=simmechanics.library.frames_transforms.rigid_transform
  Arm1 : PMIOPort  Port=1  Side=Left
  Tool1 : PMIOPort  Port=2  Side=Right
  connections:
  Tool1/RConn1 -- Rigid Transform1/RConn1
  Arm1/RConn1 -- Rigid Transform/LConn1
  Rigid Transform1/LConn1 -- Rigid Transform/RConn1 -- ForeArmCg/RConn1

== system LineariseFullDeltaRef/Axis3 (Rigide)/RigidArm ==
  ArmCG : sm_lib/Body Elements/Inertia  InertiaType=Custom  Mass=SimParam.Arm2.m  MassUnits=kg  CenterOfMass=[0 0 0]  CenterOfMassUnits=m  MomentsOfInertia=SimParam.Arm2.I'  MomentsOfInertiaUnits=kg*m^2  ProductsOfInertia=[0 0 0]  ProductsOfInertiaUnits=kg*m^2  BlockFunction=simmechanics.library.body_elements.inertia
  ArmCg-ForeArm : sm_lib/Frames and  Transforms/Rigid  Transform  TranslationMethod=Cartesian  TranslationLengthUnit=m  TranslationStandardAxis=+Z  TranslationStandardOffset=0  TranslationCartesianOffset=[SimParam.Arm2.l-SimParam.Arm2.lcg 0 0]  TranslationROffset=0  TranslationROffsetUnits=m  TranslationZOffset=0  TranslationZOffsetUnits=m  TranslationThetaOffset=0  TranslationThetaOffsetUnits=deg  RotationMethod=None  RotationAngleUnits=deg  RotationStandardAxis=+Z  RotationAngle=0  RotationArbitraryAxis=[0 0 1]  FollAlignAxisA=+X  BaseAlignAxisA=+Y  FollAlignAxisB=+Y  BaseAlignAxisB=+Z  BlockFunction=simmechanics.library.frames_transforms.rigid_transform
  ArmCg-ForeArm1 : sm_lib/Frames and  Transforms/Rigid  Transform  TranslationMethod=Cartesian  TranslationLengthUnit=m  TranslationStandardAxis=+Z  TranslationStandardOffset=0  TranslationCartesianOffset=[SimParam.Arm2.lcg 0 0]  TranslationROffset=0  TranslationROffsetUnits=m  TranslationZOffset=0  TranslationZOffsetUnits=m  TranslationThetaOffset=0  TranslationThetaOffsetUnits=deg  RotationMethod=None  RotationAngleUnits=deg  RotationStandardAxis=+Z  RotationAngle=0  RotationArbitraryAxis=[0 0 1]  FollAlignAxisA=+X  BaseAlignAxisA=+Y  FollAlignAxisB=+Y  BaseAlignAxisB=+Z  BlockFunction=simmechanics.library.frames_transforms.rigid_transform
  Motor : PMIOPort  Port=1  Side=Left
  ForeArm : PMIOPort  Port=2  Side=Right
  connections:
  ArmCg-ForeArm1/LConn1 -- Motor/RConn1
  ForeArm/RConn1 -- ArmCg-ForeArm/RConn1
  ArmCg-ForeArm1/RConn1 -- ArmCG/RConn1 -- ArmCg-ForeArm/LConn1
